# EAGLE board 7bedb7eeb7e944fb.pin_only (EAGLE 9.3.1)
REV: B

Size 25.4 x 43.69 mm. Coordinates in mm from the lower left corner, seen from the top.
Outline: 0,41.15 0,2.54 arc90 2.54,0 22.86,0 arc90 25.4,2.54 25.4,41.15 arc90 22.86,43.69 2.54,43.69 arc90 0,41.15
Copper layers (1*16): Top 0.035mm / dielectric 1.5mm / Bottom 0.035mm
Design rules "adafruit *": minimum track width 10mil, minimum drill 15.5mil, track to track 8mil, track to pad 8mil, pad to pad 8mil, via to via 8mil, smd to smd 8mil, copper to edge 10mil, drill to drill 8mil, minimum pad ring 10mil, minimum via ring 8mil, stop-mask expansion 2mil, vias tented up to drill 20mil, thermal gap 10mil

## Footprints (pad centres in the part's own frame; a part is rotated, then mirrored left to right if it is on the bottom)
0805-NO = smd 1.24 x 1.5: 1 -0.95,0; 2 0.95,0
SOD-323 = smd 1.35 x 0.8: A 1.27,0; C -1.27,0
CHIPLED_0805_NOOUTLINE = smd 1.2 x 1.2: A 0,-1.05; C 0,1.05
SOD-123 = smd 1.4 x 1.4: A 1.85,0; C -1.85,0
FIDUCIAL_1MM = smd 1 x 1: 1 0,0
1X06_ROUND_70 = drill 1 pad 1.778: 1 -6.35,0; 2 -3.81,0; 3 -1.27,0; 4 1.27,0; 5 3.81,0; 6 6.35,0
1X15_ROUND_70 = drill 1 pad 1.676: 1 -17.78,0; 2 -15.24,0; 3 -12.7,0; 4 -10.16,0; 5 -7.62,0; 6 -5.08,0; 7 -2.54,0; 8 0,0; 9 2.54,0; 10 5.08,0; 11 7.62,0; 12 10.16,0; 13 12.7,0; 14 15.24,0; 15 17.78,0
0603-NO = smd 1.075 x 1: 1 -0.85,0; 2 0.85,0
BTN_KMR2_4.6X2.8 = smd 0.9 x 0.9: A 2.05,0.8; A' -2.05,0.8; B 2.05,-0.8; B' -2.05,-0.8
SOT23-5 = smd 0.55 x 1.2: 1 -0.95,-1.3; 2 0,-1.3; 3 0.95,-1.3; 4 0.95,1.3; 5 -0.95,1.3
MOUNTINGHOLE_2.5_PLATED = drill 2.5 pad 3.2: P$1 0,0
WROOM32 = smd 1.5 x 0.9: 1 -8.6,5; 2 -8.6,3.73; 3 -8.6,2.46; 4 -8.6,1.19; 5 -8.6,-0.08; 6 -8.6,-1.35; 7 -8.6,-2.62; 8 -8.6,-3.89; 9 -8.6,-5.16; 10 -8.6,-6.43; 11 -8.6,-7.7; 12 -8.6,-8.97; 13 -8.6,-10.24; 14 -8.6,-11.51; 25 8.6,-11.51; 26 8.6,-10.24; 27 8.6,-8.97; 28 8.6,-7.7; 29 8.6,-6.43; 30 8.6,-5.16; 31 8.6,-3.89; 32 8.6,-2.62; 33 8.6,-1.35; 34 8.6,-0.08; 35 8.6,1.19; 36 8.6,2.46; 37 8.6,3.73; 38 8.6,5 | smd 0.9 x 1.5: 15 -5.7,-12.9; 16 -4.43,-12.9; 17 -3.16,-12.9; 18 -1.89,-12.9; 19 -0.62,-12.9; 20 0.65,-12.9; 21 1.92,-12.9; 22 3.19,-12.9; 23 4.46,-12.9; 24 5.73,-12.9 | smd 6 x 6: P$1 0.34,-2.7
JSTPH2 = smd 1 x 4.6: 1 -1,-3.7; 2 1,-3.7 | smd 1.6 x 3.4: NC1 -3.4,1.5; NC2 3.4,1.5

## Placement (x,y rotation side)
C1  10uF  [0805-NO]  10.54,11.05 0 top
C2  10uF  [0805-NO]  16.64,13.72 90 top
C3  10uF  [0805-NO]  13.97,13.46 0 top
C4  10uF  [0805-NO]  10.54,12.83 0 top
C5  1uF  [0805-NO]  9.53,7.37 0 top
D1  1n4148  [SOD-323]  5.71,7.37 0 top
D2  1n4148  [SOD-323]  16.38,16.13 0 top
D3  RED  [CHIPLED_0805_NOOUTLINE]  10.92,15.75 270 top
D5  MBR120  [SOD-123]  13.97,7.37 180 top
D6  MBR120  [SOD-123]  17.65,9.27 270 top
FID1  FIDUCIAL_1MM  [FIDUCIAL_1MM]  21.21,37.59 0 top
FID3  FIDUCIAL_1MM  [FIDUCIAL_1MM]  5.08,1.02 0 top
JP1  FTDI  [1X06_ROUND_70]  12.7,2.54 0 top
JP2  [1X15_ROUND_70]  1.27,23.5 270 top
JP5  [1X15_ROUND_70]  24.13,23.5 270 top
R2  1K  [0603-NO]  6.99,15.37 0 top
R4  10K  [0603-NO]  10.16,9.14 0 top
SW1  KMR2  [BTN_KMR2_4.6X2.8]  6.1,10.92 90 top
SW2  KMR2  [BTN_KMR2_4.6X2.8]  20.19,10.92 90 top
U1  AP2112-3.3  [SOT23-5]  14.48,10.54 90 top
U$2  [HUZZAHLOGO]  21.59,39.12 0 bottom
U$3  [ADAFRUIT_2.5MM]  4.06,3.81 0 top
U$12  [ADAFRUIT_TEXT_20MM]  22.86,28.19 0 bottom
U$13  [PCBFEAT-REV-040]  21.72,35.81 0 bottom
U$15  MOUNTINGHOLE2.5  [MOUNTINGHOLE_2.5_PLATED]  2.54,2.54 0 top
U$16  MOUNTINGHOLE2.5  [MOUNTINGHOLE_2.5_PLATED]  22.86,2.54 0 top
X1  ESP32_WROOM32  [WROOM32]  12.7,30.99 0 top
X2  JSTPH  [JSTPH2]  12.7,8.89 180 bottom

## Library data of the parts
C1-C5 D1-D3 D5 D6 JP1 JP2 JP5 R2 R4 SW1 SW2 U1 U$2 U$3 U$12 U$13 X1 X2 = microbuilder
FID1 FID3 U$15 U$16 = microbuilder; BOM: EXCLUDE

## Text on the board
tPlace: RST | 23 | 36 | 22 | 39 | TX | 34 | RX | 35 | 21 | 32 | 19 | 33 | 18 | 25 | #5 | 26 | 17 | 27 | 16 | 14 | #4 | 12 | Reset | #13 | GPIO0 | #0 | 13 | #2 | 3V | 15 | GND | Huzzah! ESP32 | Bat | TX | RX | V+ | GND
bPlace: ESP32 | V+: 3.5-6VDC / VBat: 3.5-6VDC / RX,RST: 5V OK | TX | RX | V+ | GND

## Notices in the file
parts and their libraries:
microbuilder: This work is placed in the public domain, and may be freely used for commercial and non-commercial work with the following conditions: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
